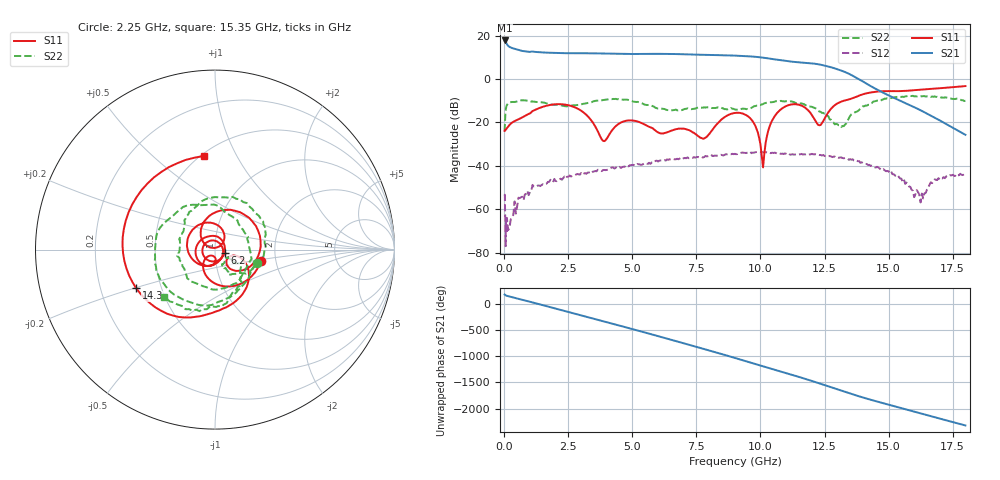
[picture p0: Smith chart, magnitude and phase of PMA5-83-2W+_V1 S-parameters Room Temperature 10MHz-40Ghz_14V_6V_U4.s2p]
!Mini-Circuits Laboratory
!S-Parameters
!Model: US-AMP-1
!Run / Lot / Date Code: N/A /  / N/A
!Fixture: ON TB-
!Network Analyzer: NFA N8975A;  Serial number: 74408
!Date: 12/1/2023 at 8:05:54 AM
!No.: Unit# 2 (#4)
!Tested with:
!Condition 4: Vdd = +14V; Vg2= +6V; Idd= 400mA
# Hz  S  dB  R  50
!Frequency  S11 dB  S11 Deg  S21 dB  S21 Deg  S12 dB  S12 Deg  S22 dB  S22 Deg
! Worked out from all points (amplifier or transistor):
!   368 points, 10 MHz to 18 GHz, reference 50 ohm
!   highest |S21| = 17.8 dB at 20 MHz (marker M1)
!   |S21| within 3 dB of that: start of sweep to 205.2 MHz
!   unconditionally stable (mu >= 1): start of sweep to end of sweep
!   at 2.7 GHz: K = 19.06, MAG = 12.4 dB, |S12| = -44.5 dB
!   at 8.85 GHz: K = 7.28, MAG = 11.1 dB, |S12| = -34.7 dB
!   at 18 GHz: K = 707.24, MAG = -22.5 dB, |S12| = -43.8 dB
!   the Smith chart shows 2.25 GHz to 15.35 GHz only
!   S11 on the Smith chart (normalised r, x): 2.25 GHz: 1.66, -0.23; 6.2 GHz: 1.11, -0.04; 14.3 GHz: 0.36, -0.20; 15.35 GHz: 0.52, +0.74
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1e7  -23.87 -0.2  17.59 177.2  -53.65 -35.9  -24.03 -71.6
2e7  -23.62 -3.8  17.76 173.9  -53.29 131.3  -20.83 -90.6
5e8  -18.84 -146.1  13.57 101.2  -58.61 31.2  -10.30 139.7
1.15e9  -14.47 113.8  12.54 20.3  -49.54 -41.7  -10.44 66.5
2.25e9  -11.63 -14.6  11.91 -120.7  -46.41 178.0  -12.25 -18.4
3.05e9  -15.03 -96.7  11.86 135.3  -44.05 79.7  -11.51 -63.0
4e9  -27.43 -91.7  11.70 9.8  -41.87 -40.0  -9.41 -132.0
4.75e9  -19.24 -134.1  11.53 -88.9  -40.82 -135.1  -9.49 164.9
5.4e9  -20.52 145.7  11.55 -174.9  -39.34 144.2  -11.34 112.8
6.05e9  -24.86 18.4  11.59 97.3  -37.64 61.0  -13.62 63.6
6.2e9  -25.09 -16.9  11.57 76.8  -37.54 40.5  -13.73 54.4
7.4e9  -24.80 122.2  11.24 -87.7  -35.96 -114.3  -13.78 -38.5
8.15e9  -22.94 -75.7  11.04 168.7  -35.51 144.3  -13.36 -108.3
9.05e9  -15.59 144.7  10.76 41.4  -34.64 25.1  -14.11 177.9
9.85e9  -23.10 45.2  10.17 -75.4  -33.64 -87.9  -12.25 131.3
1.05e10  -18.16 130.1  9.14 -170.6  -34.09 -176.9  -10.59 80.8
1.12e10  -11.70 42.7  8.03 89.0  -34.80 88.5  -10.27 22.7
1.205e10  -17.32 -51.9  7.15 -38.4  -34.65 -34.3  -13.02 -34.7
1.43e10  -6.21 -153.8  -3.25 -30.2  -40.03 -28.2  -11.29 -71.8
1.505e10  -5.57 130.3  -7.82 -130.8  -43.29 -112.1  -8.62 -116.3
1.535e10  -5.59 96.9  -9.50 -170.4  -44.07 -145.7  -8.20 -137.2
1.8e10  -3.27 159.8  -25.71 -161.0  -43.76 49.8  -10.01 46.1
